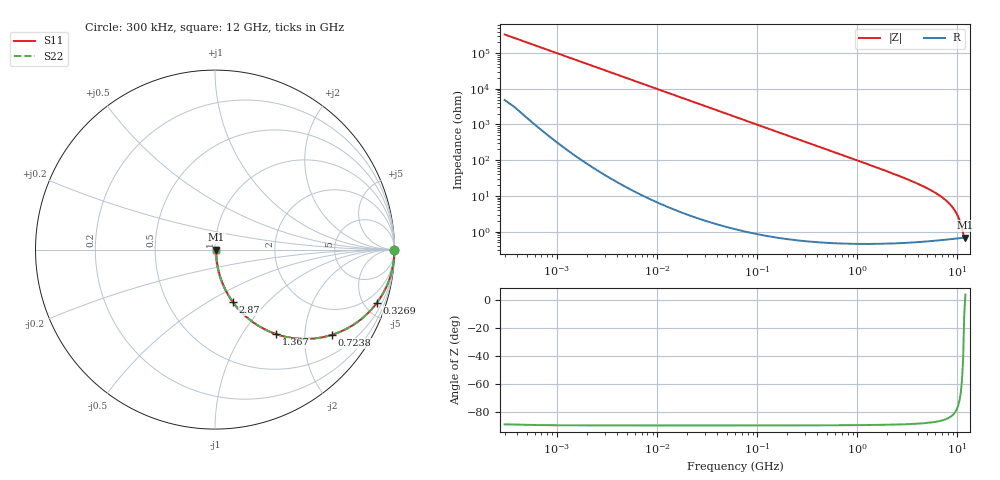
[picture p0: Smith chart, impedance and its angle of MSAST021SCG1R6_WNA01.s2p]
! MSAST021SCG1R6_WNA01  S-PARAMETER MODEL  ( General Type )
! Model Generated by TAIYO YUDEN Corporation (http://www.ty-top.com)
! Version 2.0
! TAIYO YUDEN Control No. 181101
! Copyright(c) 2015 TAIYO YUDEN CO.,LTD. All Rights Reserved.
! Product Description (link to TY-COMPAS)
! https://ds.yuden.co.jp/TYCOMPAS/or/detail?pn=MSAST021SCG1R6BWNA01&u=M
! Products Name : Multilayer Ceramic Capacitors
! Characteristics :
!  Capacitance : 1.6 pF , Rated Voltage : 25V , TCC : CG / C0G
!  Case Size : 0.25 x 0.125 / 0.0098 x 0.0049 [mm/inch] , Thickness : 0.125 / 0.0049 [mm/inch]
!  (Conditions: Temperature = 25 degC , DC Bias Current/Voltage = 0A / 0V)
! External Node Assignments :
!  1  o---| |---o  2
! GND o---------o GND
! Frequency Range : 0.3MHz  -  12000MHz  [ 401 STEP ]
# MHz S RI R 50
! Freq[MHz].  S11 Real  S11 Imag  S21 Real  S21 Imag  S12 Real  S12 Imag  S22 Real  S22 Imag
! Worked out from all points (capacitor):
!   401 points, 300 kHz to 12 GHz, reference 50 ohm
!   read as one part in series: C = 1.6 pF near 316.3 kHz
!   lowest |Z| = 684 mohm at 12 GHz (marker M1)
!   series resonance near 11.91 GHz, so ESL is about 110 pH
!   S11 on the Smith chart (normalised r, x): 300 kHz: open; 326.9 MHz: 1.01, -6.08; 723.8 MHz: 1.01, -2.74; 1.367 GHz: 1.01, -1.44; 2.87 GHz: 1.01, -0.65; 12 GHz: 1.01, +0.00
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0.3  1 -0.000302  4.49e-06 0.000302  4.49e-06 0.000302  1 -0.000302
1.769972  1 -0.00178  6.31e-06 0.00178  6.31e-06 0.00178  1 -0.00178
10.44266  0.9999 -0.0105  0.000117 0.0105  0.000117 0.0105  0.9999 -0.0105
60  0.9963 -0.0601  0.00367 0.0601  0.00367 0.0601  0.9963 -0.0601
147.6816  0.9783 -0.1452  0.0217 0.1452  0.0217 0.1452  0.9783 -0.1452
326.9496  0.9019 -0.2965  0.0981 0.2965  0.0981 0.2965  0.9019 -0.2965
353.9943  0.887 -0.3157  0.113 0.3157  0.113 0.3157  0.887 -0.3157
512.9422  0.7887 -0.407  0.2113 0.407  0.2113 0.407  0.7887 -0.407
723.8279  0.6516 -0.4748  0.3484 0.4748  0.3484 0.4748  0.6516 -0.4748
994.7115  0.4965 -0.4977  0.5035 0.4977  0.5035 0.4977  0.4965 -0.4977
1366.97  0.3411 -0.4709  0.6589 0.4709  0.6589 0.4709  0.3411 -0.4709
2088.533  0.178 -0.3775  0.822 0.3775  0.822 0.3775  0.178 -0.3775
2870.14  0.0996 -0.2922  0.9004 0.2922  0.9004 0.2922  0.0996 -0.2922
4050.141  0.0493 -0.205  0.9507 0.205  0.9507 0.205  0.0493 -0.205
5278.635  0.0272 -0.1459  0.9728 0.1459  0.9728 0.1459  0.0272 -0.1459
6524.734  0.0166 -0.1035  0.9834 0.1035  0.9834 0.1035  0.0166 -0.1035
7854.144  0.0108 -0.0694  0.9892 0.0694  0.9892 0.0694  0.0108 -0.0694
8732.115  0.00876 -0.0508  0.9912 0.0508  0.9912 0.0508  0.00876 -0.0508
9708.23  0.00743 -0.0327  0.9926 0.0327  0.9926 0.0327  0.00743 -0.0327
10511.28  0.00688 -0.0194  0.9931 0.0194  0.9931 0.0194  0.00688 -0.0194
11380.75  0.0067 -0.00621  0.9933 0.00621  0.9933 0.00621  0.0067 -0.00621
12000  0.00677 0.00049  0.9932 -0.00049  0.9932 -0.00049  0.00677 0.00049
